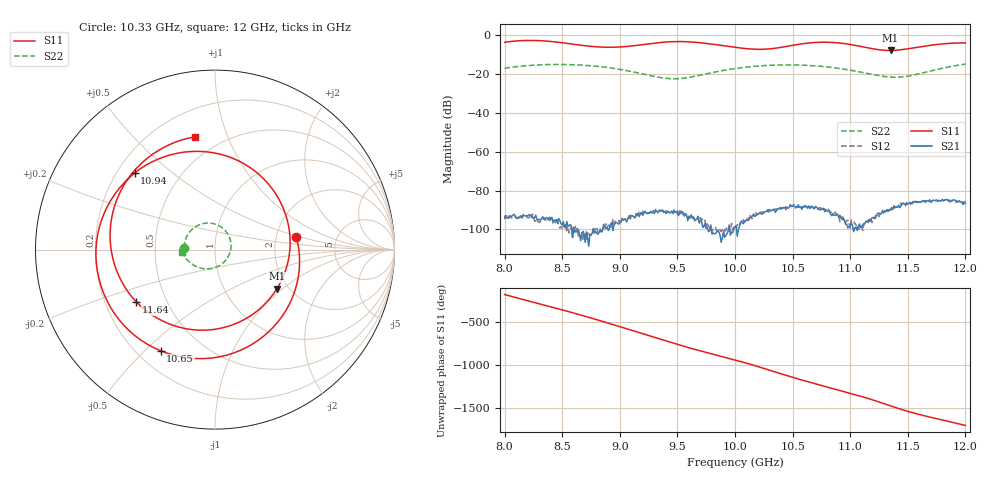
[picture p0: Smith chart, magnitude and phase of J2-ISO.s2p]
!Keysight Technologies,N5234A,MY52241180,A.10.60.03
!Date: Tuesday, May 30, 2023 15:18:08
!Correction: S11(Full 2 Port(1,2))
!S21(Full 2 Port(1,2))
!S12(Full 2 Port(1,2))
!S22(Full 2 Port(1,2))
!S2P File: Measurements: S11, S21, S12, S22:
# Hz S  dB  R 50
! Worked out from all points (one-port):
!   401 points, 8 GHz to 12 GHz, reference 50 ohm
!   lowest |S11| = -7.8 dB at 11.35 GHz (marker M1), VSWR 2.38, Z = 87.3 - j45.8 ohm
!   |S11| at or under -10 dB: nowhere
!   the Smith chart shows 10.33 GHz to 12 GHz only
!   S11 on the Smith chart (normalised r, x): 10.33 GHz: 2.59, +0.47; 10.65 GHz: 0.29, -0.56; 10.94 GHz: 0.27, +0.38; 11.64 GHz: 0.34, -0.27; 12 GHz: 0.36, +0.77
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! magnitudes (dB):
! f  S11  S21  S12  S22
! 8 GHz  -3.6  -93.2  -94.8  -17.0
! 8.15 GHz  -2.7  -94.0  -94.1  -15.8
! 8.29 GHz  -2.7  -95.1  -95.9  -15.2
! 8.67 GHz  -5.1  -101.9  -102.4  -15.3
! 8.96 GHz  -6.1  -97.0  -95.8  -17.1
! 9.34 GHz  -3.8  -90.6  -90.1  -21.6
! 9.45 GHz  -3.3  -90.5  -90.8  -22.4
! 9.55 GHz  -3.2  -91.4  -92.0  -22.1
! 10 GHz  -6.2  -98.7  -97.9  -17.1
! 10.18 GHz  -7.2  -92.7  -91.2  -15.9
! 10.33 GHz  -6.8  -90.0  -89.7  -15.4
! 10.65 GHz  -3.9  -89.2  -88.7  -15.5
! 10.67 GHz  -3.8  -88.1  -88.7  -15.6
! 10.81 GHz  -3.5  -90.6  -89.6  -16.3
! 10.94 GHz  -4.2  -95.1  -93.8  -17.4
! 11.23 GHz  -7.2  -92.6  -92.3  -20.5
! 11.34 GHz  -7.8  -89.8  -89.9  -21.5
! 11.35 GHz  -7.8  -89.7  -90.0  -21.5
! 11.48 GHz  -7.1  -87.3  -87.8  -21.2
! 11.64 GHz  -5.6  -85.3  -85.4  -19.2
! 11.83 GHz  -4.3  -84.7  -84.7  -16.6
! 12 GHz  -3.9  -86.7  -85.8  -14.8
